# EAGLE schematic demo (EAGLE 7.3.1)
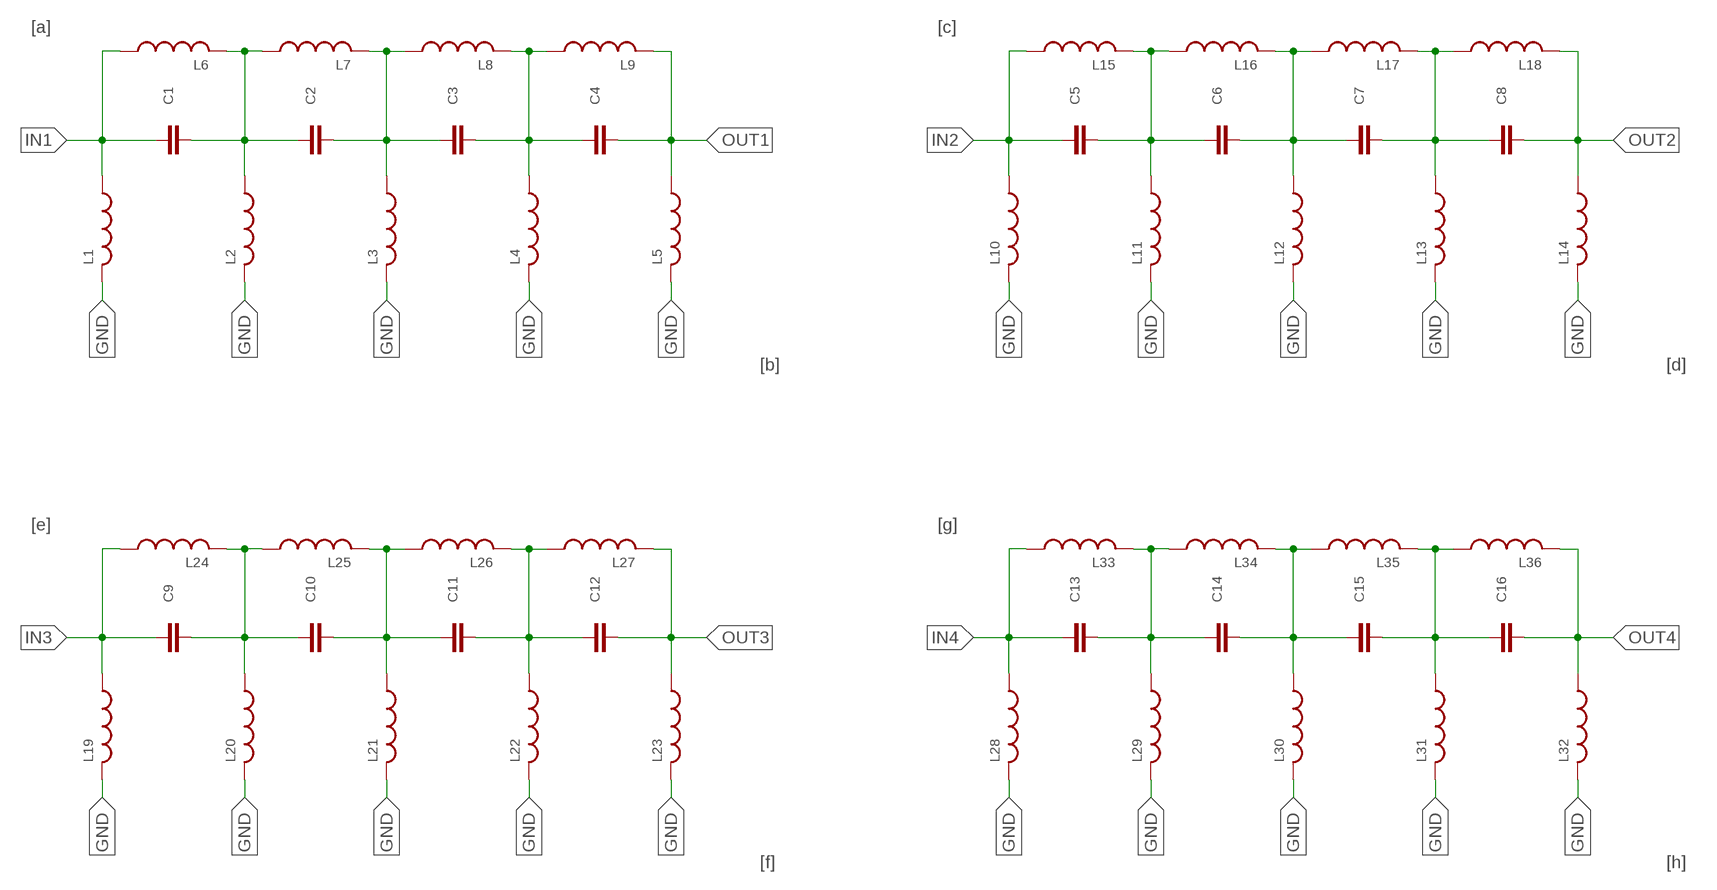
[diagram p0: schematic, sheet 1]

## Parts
C1  LTDB_PASSIVES_CAP-NP-SMT-C0402  [LTDB_PASSIVES_C0402]
C2  LTDB_PASSIVES_CAP-NP-SMT-C0402  [LTDB_PASSIVES_C0402]
C3  LTDB_PASSIVES_CAP-NP-SMT-C0402  [LTDB_PASSIVES_C0402]
C4  LTDB_PASSIVES_CAP-NP-SMT-C0402  [LTDB_PASSIVES_C0402]
C5  LTDB_PASSIVES_CAP-NP-SMT-C0402  [LTDB_PASSIVES_C0402]
C6  LTDB_PASSIVES_CAP-NP-SMT-C0402  [LTDB_PASSIVES_C0402]
C7  LTDB_PASSIVES_CAP-NP-SMT-C0402  [LTDB_PASSIVES_C0402]
C8  LTDB_PASSIVES_CAP-NP-SMT-C0402  [LTDB_PASSIVES_C0402]
C9  LTDB_PASSIVES_CAP-NP-SMT-C0402  [LTDB_PASSIVES_C0402]
C10  LTDB_PASSIVES_CAP-NP-SMT-C0402  [LTDB_PASSIVES_C0402]
C11  LTDB_PASSIVES_CAP-NP-SMT-C0402  [LTDB_PASSIVES_C0402]
C12  LTDB_PASSIVES_CAP-NP-SMT-C0402  [LTDB_PASSIVES_C0402]
C13  LTDB_PASSIVES_CAP-NP-SMT-C0402  [LTDB_PASSIVES_C0402]
C14  LTDB_PASSIVES_CAP-NP-SMT-C0402  [LTDB_PASSIVES_C0402]
C15  LTDB_PASSIVES_CAP-NP-SMT-C0402  [LTDB_PASSIVES_C0402]
C16  LTDB_PASSIVES_CAP-NP-SMT-C0402  [LTDB_PASSIVES_C0402]
L1  L-US0402  [LTDB_PASSIVES_R0402]
L2  L-US0402  [LTDB_PASSIVES_R0402]
L3  L-US0402  [LTDB_PASSIVES_R0402]
L4  L-US0402  [LTDB_PASSIVES_R0402]
L5  L-US0402  [LTDB_PASSIVES_R0402]
L6  L-US0402  [LTDB_PASSIVES_R0402]
L7  L-US0402  [LTDB_PASSIVES_R0402]
L8  L-US0402  [LTDB_PASSIVES_R0402]
L9  L-US0402  [LTDB_PASSIVES_R0402]
L10  L-US0402  [LTDB_PASSIVES_R0402]
L11  L-US0402  [LTDB_PASSIVES_R0402]
L12  L-US0402  [LTDB_PASSIVES_R0402]
L13  L-US0402  [LTDB_PASSIVES_R0402]
L14  L-US0402  [LTDB_PASSIVES_R0402]
L15  L-US0402  [LTDB_PASSIVES_R0402]
L16  L-US0402  [LTDB_PASSIVES_R0402]
L17  L-US0402  [LTDB_PASSIVES_R0402]
L18  L-US0402  [LTDB_PASSIVES_R0402]
L19  L-US0402  [LTDB_PASSIVES_R0402]
L20  L-US0402  [LTDB_PASSIVES_R0402]
L21  L-US0402  [LTDB_PASSIVES_R0402]
L22  L-US0402  [LTDB_PASSIVES_R0402]
L23  L-US0402  [LTDB_PASSIVES_R0402]
L24  L-US0402  [LTDB_PASSIVES_R0402]
L25  L-US0402  [LTDB_PASSIVES_R0402]
L26  L-US0402  [LTDB_PASSIVES_R0402]
L27  L-US0402  [LTDB_PASSIVES_R0402]
L28  L-US0402  [LTDB_PASSIVES_R0402]
L29  L-US0402  [LTDB_PASSIVES_R0402]
L30  L-US0402  [LTDB_PASSIVES_R0402]
L31  L-US0402  [LTDB_PASSIVES_R0402]
L32  L-US0402  [LTDB_PASSIVES_R0402]
L33  L-US0402  [LTDB_PASSIVES_R0402]
L34  L-US0402  [LTDB_PASSIVES_R0402]
L35  L-US0402  [LTDB_PASSIVES_R0402]
L36  L-US0402  [LTDB_PASSIVES_R0402]

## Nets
GND: L1.2 L2.2 L3.2 L4.2 L5.2 L10.2 L11.2 L12.2 L13.2 L14.2 L19.2 L20.2 L21.2 L22.2 L23.2 L28.2 L29.2 L30.2 L31.2 L32.2
IN1: C1.1 L1.1 L6.1
IN2: C5.1 L10.1 L15.1
IN3: C9.1 L19.1 L24.1
IN4: C13.1 L28.1 L33.1
N$1: C5.2 C6.1 L11.1 L15.2 L16.1
N$2: C6.2 C7.1 L12.1 L16.2 L17.1
N$3: C7.2 C8.1 L13.1 L17.2 L18.1
N$4: C9.2 C10.1 L20.1 L24.2 L25.1
N$5: C10.2 C11.1 L21.1 L25.2 L26.1
N$6: C11.2 C12.1 L22.1 L26.2 L27.1
N$7: C13.2 C14.1 L29.1 L33.2 L34.1
N$8: C14.2 C15.1 L30.1 L34.2 L35.1
N$9: C15.2 C16.1 L31.1 L35.2 L36.1
N$20: C1.2 C2.1 L2.1 L6.2 L7.1
N$21: C2.2 C3.1 L3.1 L7.2 L8.1
N$22: C3.2 C4.1 L4.1 L8.2 L9.1
OUT1: C4.2 L5.1 L9.2
OUT2: C8.2 L14.1 L18.2
OUT3: C12.2 L23.1 L27.2
OUT4: C16.2 L32.1 L36.2

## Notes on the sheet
- [a] | [c]
- [b] | [d]
- [e] | [g]
- [f] | [h]

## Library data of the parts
C1-C16 = vnatest:LTDB_PASSIVES_CAP-NP-SMT-: Capacitor; Non-polar; SMT
L1-L36 = vnatest:L-US: INDUCTOR, American symbol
